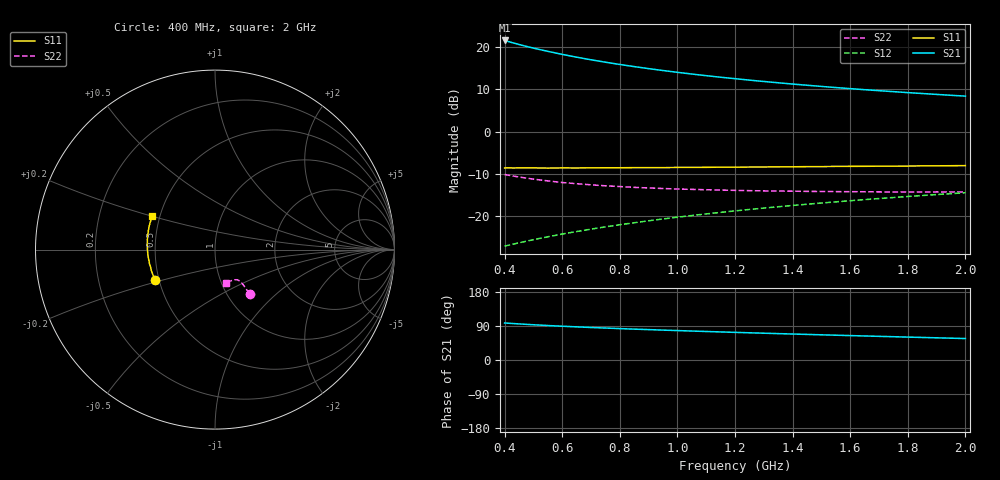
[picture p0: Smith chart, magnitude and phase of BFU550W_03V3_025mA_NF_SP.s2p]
! Filename:  P:\Prog\Test\Noise\ATS_data\Testdata_Net\06 Compressed Noise after Statistics\BFU550W_APM2013_11_D05_03p3V_025mA_NF_CM01_D.sf
! Date/Time: Tue 26/Mar/2013 16:25:21
! BFU550W_APM2013_11_D05_03p3V_1to35mA_NF_CM01_Bias8_R.sf
! Noise Parameter Data File
! BFU550W_APM2013_11_D05_03p3V_1to35mA_NF_CM01
! Date/time: Mon Mar 25 12:16:07 2013
! VAR V_out= 3.301000
! VAR I_out= 25.000000
! VAR V_in= 0.841600
! VAR I_in= 0.272950
! Device data file deembeded for feedlines and parallel
! Original file: \06 Compressed Noise after Statistics\BFU550W_APM2013_11_D05_03p3V_025mA_NF_CM01_R.sf
! Feed-files: PR019V01_070313_Feed1.s2p, PR019V01_070313_Feed2.s2p
! Parallel-file: PR019V01_070313_Par.s2p
# MHz S MA R 50
!  Freq-MHz  S11-mag  S11-arg  S21-mag  S21-arg  S12-mag  S12-arg  S22-mag  S22-arg
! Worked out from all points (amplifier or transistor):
!   37 points, 400 MHz to 2 GHz, reference 50 ohm
!   highest |S21| = 21.5 dB at 400 MHz (marker M1)
!   |S21| within 3 dB of that: start of sweep to 580.1 MHz
!   unconditionally stable (mu >= 1): 861.2 MHz to end of sweep
!   at 500 MHz: K = 0.93, MSG = 22.6 dB, |S12| = -25.5 dB
!   at 1.1 GHz: K = 1.01, MAG = 15.6 dB, |S12| = -19.4 dB
!   at 2 GHz: K = 1.00, MAG = 11.1 dB, |S12| = -14.4 dB
!   lowest NFmin = 1.02 dB at 420 MHz
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400  0.373 -153.4  11.93 97.8  0.0445 67.7  0.3122 -51.7
420  0.3734 -155.3  11.4 96.7  0.04622 68.1  0.3037 -51.7
440  0.3733 -157.0  10.92 95.7  0.04793 68.4  0.2954 -51.6
460  0.3732 -158.5  10.48 94.8  0.04962 68.7  0.2881 -51.6
480  0.3731 -160.1  10.07 93.9  0.05136 69.0  0.2816 -51.7
500  0.3735 -161.6  9.691 93.0  0.05303 69.2  0.2753 -51.5
550  0.3717 -164.8  8.877 91.0  0.05744 69.8  0.2623 -51.4
600  0.3734 -167.7  8.173 89.1  0.06182 70.2  0.2511 -51.2
650  0.3728 -170.3  7.574 87.4  0.06624 70.6  0.2431 -51.3
700  0.374 -172.7  7.056 85.8  0.07072 70.9  0.2357 -51.4
750  0.3749 -174.8  6.607 84.3  0.07517 71.1  0.2295 -51.5
800  0.3748 -176.9  6.211 82.9  0.07966 71.2  0.2249 -52.0
850  0.3763 -178.9  5.862 81.5  0.08412 71.3  0.22 -52.1
950  0.3765 177.7  5.269 78.9  0.09323 71.4  0.2133 -52.8
1050  0.3784 174.5  4.79 76.4  0.1023 71.3  0.2083 -53.9
1150  0.3813 171.4  4.391 74.1  0.1114 71.1  0.2044 -55.2
1200  0.3812 170.1  4.221 72.9  0.1161 70.9  0.2029 -56.0
1350  0.3838 166.2  3.776 69.6  0.1299 70.3  0.1988 -58.1
1500  0.3869 162.5  3.421 66.5  0.1438 69.5  0.197 -60.9
1650  0.3901 158.9  3.131 63.4  0.1577 68.7  0.1953 -63.6
1750  0.3918 156.9  2.967 61.4  0.167 68.1  0.1942 -65.7
2000  0.398 151.6  2.628 56.6  0.1902 66.4  0.1944 -71.5
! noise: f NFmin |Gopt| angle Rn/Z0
400  1.025  0.3675  -171.1  0.0604
460  1.032  0.3694  -168.8  0.0622
600  1.106  0.3666  -167.2  0.0631
800  1.073  0.3912  -163.7  0.0627
1000  1.111  0.4069  -160.2  0.0618
1200  1.124  0.4103  -155.6  0.0699
1400  1.187  0.4351  -152.7  0.068
1600  1.2  0.4429  -148.6  0.076
1800  1.237  0.4533  -144.3  0.0859
2000  1.272  0.4437  -141.4  0.0982
